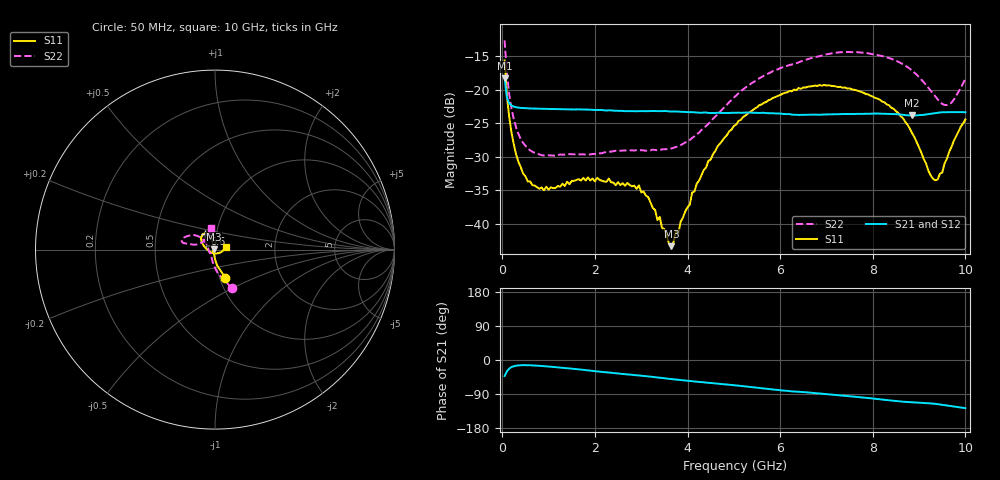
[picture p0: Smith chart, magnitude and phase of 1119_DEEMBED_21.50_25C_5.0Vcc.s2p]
!Hittite Microwave Corp.
!Digital Attenuator/PhaseShifter Rev 1.4.0
!Filename: C:\DATA\DATA\1119_DEEMBED_21.50_25C_5.0Vcc.s2p
!VNA ID: Agilent Technologies,N5224A,MY51441122,A.10.45.03
!Device type:
!2 Port Calibration.
!Temp(C): 25
!Lot Number:
!Serial Number:
!Operator:
!Misc:
!Attenuator:  21.500
# GHZ S DB R 50.0
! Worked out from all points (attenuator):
!   200 points, 50 MHz to 10 GHz, reference 50 ohm
!   highest |S21| = -18.24 dB at 50 MHz (marker M1); lowest = -23.8 dB at 8.85 GHz (marker M2)
!   lowest |S11| = -43.4 dB at 3.65 GHz (marker M3), VSWR 1.01, Z = 49.3 + j0.134 ohm
!   |S11| at or under -10 dB: start of sweep to end of sweep
!   |S22| runs from -29.8 to -12.6 dB; largest |S21 - S12| = 0.00024
!   S11 on the Smith chart (normalised r, x): 50 MHz: 1.06, -0.34; 6.6 GHz: 0.88, +0.16; 10 GHz: 1.12, +0.03
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0.05  -15.59 -70.0  -18.24 -42.3  -18.24 -42.3  -12.60 -66.5
0.1  -20.88 -81.8  -21.18 -29.8  -21.17 -29.8  -17.55 -83.4
0.2  -26.45 -91.6  -22.34 -18.6  -22.34 -18.6  -22.84 -100.1
0.35  -30.79 -99.4  -22.65 -14.2  -22.65 -14.2  -26.62 -114.1
0.55  -33.69 -108.3  -22.76 -13.7  -22.76 -13.7  -28.71 -125.7
0.9  -35.04 -116.6  -22.83 -16.2  -22.84 -16.2  -29.82 -135.0
1.75  -33.16 -126.9  -22.94 -26.1  -22.94 -26.1  -29.66 -139.7
2.95  -34.29 -122.8  -23.17 -40.8  -23.17 -40.8  -29.04 -158.7
3.35  -39.49 -136.1  -23.18 -46.1  -23.19 -46.2  -29.04 -170.6
3.4  -39.02 -146.5  -23.18 -46.7  -23.18 -46.7  -28.98 -172.0
3.65  -43.39 168.5  -23.24 -50.1  -23.25 -50.1  -28.77 179.0
4.45  -30.63 97.7  -23.45 -60.3  -23.46 -60.4  -25.08 147.5
5.05  -25.21 102.0  -23.42 -67.1  -23.44 -67.2  -20.84 139.6
5.75  -21.54 111.1  -23.49 -76.5  -23.50 -76.5  -17.52 143.8
6.6  -19.52 122.4  -23.72 -85.6  -23.73 -85.6  -15.39 153.4
6.7  -19.44 124.1  -23.70 -86.7  -23.71 -86.7  -15.18 154.5
7.5  -19.77 139.0  -23.61 -95.7  -23.62 -95.7  -14.33 163.9
8.35  -22.29 154.9  -23.60 -106.3  -23.60 -106.3  -15.23 168.0
8.85  -26.49 174.8  -23.83 -111.5  -23.83 -111.5  -17.13 167.7
9.35  -33.53 -98.0  -23.48 -115.8  -23.50 -115.8  -20.97 157.0
9.65  -29.27 -27.0  -23.33 -120.8  -23.34 -120.9  -22.16 127.0
10  -24.42 12.5  -23.35 -127.2  -23.35 -127.1  -18.36 99.5
